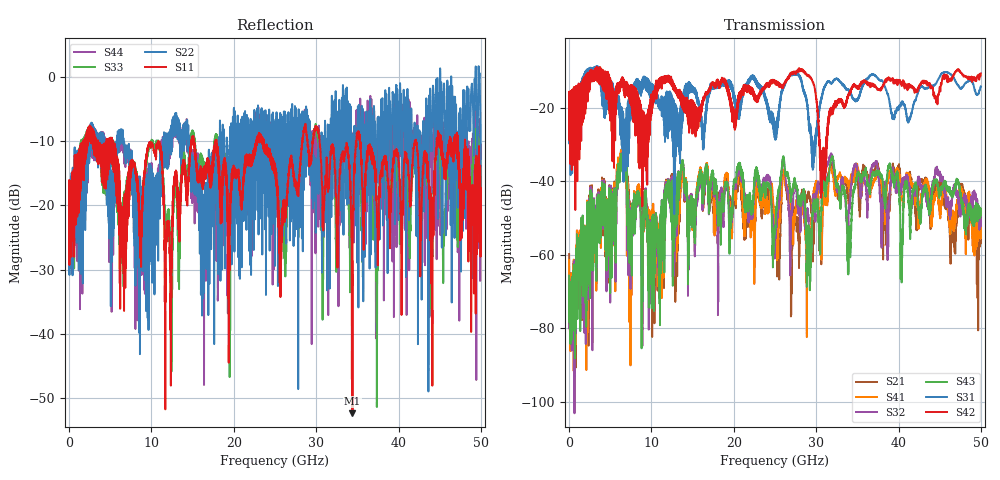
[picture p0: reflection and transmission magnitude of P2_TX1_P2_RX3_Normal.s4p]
!Keysight Technologies,N5225B,MY57041031,A.13.20.10
!Date: Friday, May 31, 2019 11:30:41
!Correction: S11(Full 4 Port(1,2,3,4))
!S12(Full 4 Port(1,2,3,4))
!S13(Full 4 Port(1,2,3,4))
!S14(Full 4 Port(1,2,3,4))
!S21(Full 4 Port(1,2,3,4))
!S22(Full 4 Port(1,2,3,4))
!S23(Full 4 Port(1,2,3,4))
!S24(Full 4 Port(1,2,3,4))
!S31(Full 4 Port(1,2,3,4))
!S32(Full 4 Port(1,2,3,4))
!S33(Full 4 Port(1,2,3,4))
!S34(Full 4 Port(1,2,3,4))
!S41(Full 4 Port(1,2,3,4))
!S42(Full 4 Port(1,2,3,4))
!S43(Full 4 Port(1,2,3,4))
!S44(Full 4 Port(1,2,3,4))
!S4P File: Measurements: <S11,S12,S13,S14>,
!<S21,S22,S23,S24>,
!<S31,S32,S33,S34>,
!<S41,S42,S43,S44>:
# Hz S  dB  R 50.0
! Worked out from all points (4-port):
!   5000 points, 10 MHz to 50 GHz, reference 50 ohm
!   strongest paths, dB at 10 MHz, 12.51 GHz, 25.01 GHz, 37.51 GHz, 50 GHz:
!     S42: -19.4, -14.0, -12.9, -15.0, -10.7
!     S31: -19.5, -17.3, -28.7, -12.1, -14.3
!     S43: -65.7, -48.2, -53.1, -37.4, -49.3
!     S32: -80.0, -46.7, -56.9, -37.2, -50.0
!     S41: -61.4, -45.7, -50.5, -37.6, -51.0
!     S21: -59.9, -44.4, -59.4, -35.8, -55.2
!   lowest |S11| = -52.3 dB at 34.41 GHz (marker M1), VSWR 1.00, Z = 50.2 + j0.152 ohm
!   |S11| at or under -10 dB: 5.36 GHz to 10.81 GHz (5.449 GHz wide, 67.4 % of centre); 17.89 GHz to 22.7 GHz (4.804 GHz wide, 23.7 % of centre); 35.31 GHz to 41.96 GHz (6.646 GHz wide, 17.2 % of centre)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
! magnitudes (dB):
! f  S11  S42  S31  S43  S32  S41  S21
! 10 MHz  -19.5  -19.4  -19.5  -65.7  -80.0  -61.4  -59.9
! 6.6 GHz  -20.3  -14.1  -28.9  -34.1  -33.5  -32.4  -32.1
! 10.12 GHz  -10.5  -20.2  -15.9  -49.6  -51.1  -47.6  -50.3
! 28.29 GHz  -11.0  -9.6  -13.3  -44.4  -45.3  -48.1  -42.3
! 30.78 GHz  -22.6  -33.2  -16.4  -41.1  -39.7  -48.3  -48.2
! 34.41 GHz  -52.3  -14.2  -17.3  -45.6  -38.1  -39.0  -38.3
! 50 GHz  -17.3  -10.7  -14.3  -49.3  -50.0  -51.0  -55.2
